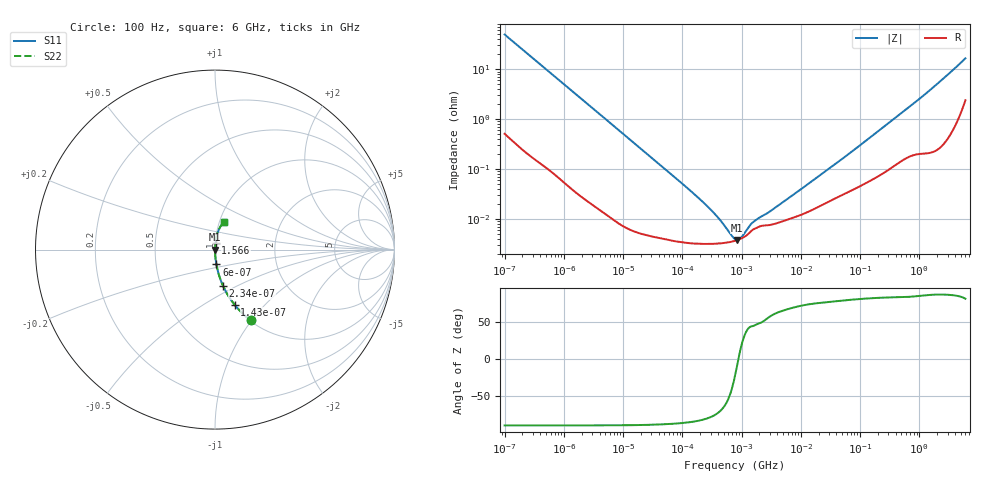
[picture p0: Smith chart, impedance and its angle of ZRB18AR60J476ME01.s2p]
!Murata Part Number: ZRB18AR60J476ME01
!These Parameters are Measured in Series Mode Connection
!Data Generated on Jun 10, 2025
!  o--ll--o
!Port1  Port2
!  o------o
!Operation Temp=25[degC], DC Bias Voltage=0[V]
!Freq. Start=100[Hz] Stop=6[GHz] 401[Steps]
# Hz S RI R 50
!Freq.(Hz) S11(Real) S11(Imag) S21(Real) S21(Imag) S12(Real) S12(Imag) S22(Real) S22(Imag)
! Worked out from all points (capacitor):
!   401 points, 100 Hz to 6 GHz, reference 50 ohm
!   read as one part in series: C = 32 uF near 109 Hz
!   lowest |Z| = 3.84 mohm at 847.2 kHz (marker M1)
!   series resonance near 883 kHz, so ESL is about 1 nH
!   S11 on the Smith chart (normalised r, x): 100 Hz: 1.01, -0.99; 143 Hz: 1.01, -0.70; 234 Hz: 1.00, -0.43; 600 Hz: 1.00, -0.17; 1.566 GHz: 1.00, +0.08; 6 GHz: 1.05, +0.33
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100  0.2 -0.3949  0.8 0.3949  0.8 0.3949  0.2 -0.3949
143  0.1103 -0.3082  0.8897 0.3082  0.8897 0.3082  0.1103 -0.3082
234  0.0452 -0.203  0.9548 0.203  0.9548 0.203  0.0452 -0.203
366  0.0196 -0.1336  0.9804 0.1336  0.9804 0.1336  0.0196 -0.1336
600  0.00785 -0.083  0.9922 0.083  0.9922 0.083  0.00785 -0.083
2008  0.000909 -0.0252  0.9991 0.0252  0.9991 0.0252  0.000909 -0.0252
40335  4.35e-05 -0.00127  1 0.00127  1 0.00127  4.35e-05 -0.00127
176758  3.23e-05 -0.000282  1 0.000282  1 0.000282  3.23e-05 -0.000282
413847  3.26e-05 -9.76e-05  1 9.76e-05  1 9.76e-05  3.26e-05 -9.76e-05
473344  3.31e-05 -7.79e-05  1 7.79e-05  1 7.79e-05  3.31e-05 -7.79e-05
774597  3.69e-05 -1.53e-05  1 1.53e-05  1 1.53e-05  3.69e-05 -1.53e-05
847162  3.81e-05 -4.8e-06  1 4.8e-06  1 4.8e-06  3.81e-05 -4.8e-06
1658239  6.41e-05 6.57e-05  0.9999 -6.57e-05  0.9999 -6.57e-05  6.41e-05 6.57e-05
1983483  7.09e-05 7.99e-05  0.9999 -7.99e-05  0.9999 -7.99e-05  7.09e-05 7.99e-05
2967816  7.62e-05 0.000119  0.9999 -0.000119  0.9999 -0.000119  7.62e-05 0.000119
1.555665e7  0.000153 0.000561  0.9998 -0.000561  0.9998 -0.000561  0.000153 0.000561
6.518806e7  0.000357 0.00201  0.9996 -0.00201  0.9996 -0.00201  0.000357 0.00201
3.124326e8  0.00107 0.00859  0.9989 -0.00859  0.9989 -0.00859  0.00107 0.00859
1.565993e9  0.00368 0.0393  0.9963 -0.0393  0.9963 -0.0393  0.00368 0.0393
3.065283e9  0.0103 0.0778  0.9897 -0.0778  0.9897 -0.0778  0.0103 0.0778
5.486059e9  0.0377 0.14  0.9623 -0.14  0.9623 -0.14  0.0377 0.14
6e9  0.0478 0.1522  0.9522 -0.1522  0.9522 -0.1522  0.0478 0.1522
